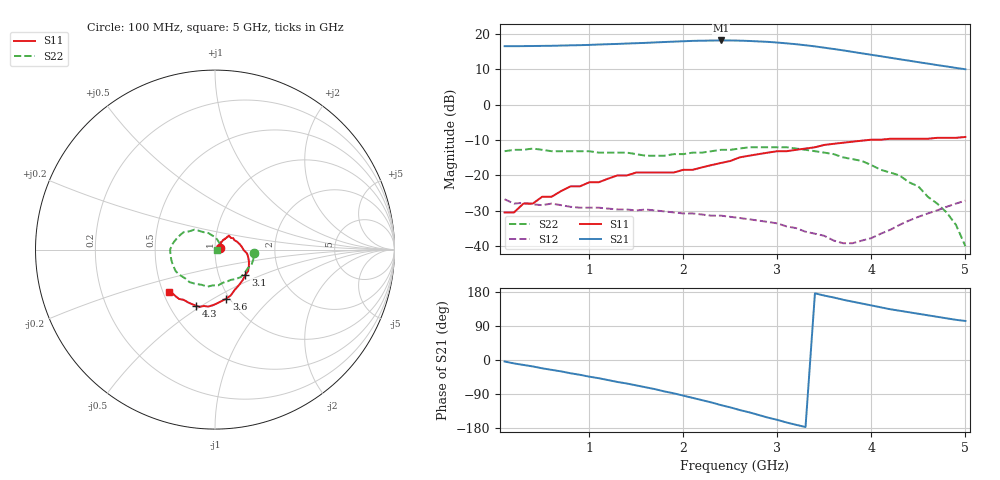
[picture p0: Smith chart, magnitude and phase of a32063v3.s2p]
!  INA-32063  S PARAMETERS
!  Vd = 3 V  LAST UPDATED 04-16-98
# ghz s ma r 50
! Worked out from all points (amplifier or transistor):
!   50 points, 100 MHz to 5 GHz, reference 50 ohm
!   highest |S21| = 18.2 dB at 2.4 GHz (marker M1)
!   |S21| within 3 dB of that: start of sweep to 3.747 GHz
!   unconditionally stable (mu >= 1): start of sweep to end of sweep
!   at 900 MHz: K = 2.07, MAG = 17.1 dB, |S12| = -29.1 dB
!   at 2.6 GHz: K = 2.33, MAG = 18.6 dB, |S12| = -32.0 dB
!   at 5 GHz: K = 3.21, MAG = 10.6 dB, |S12| = -27.1 dB
!   S11 on the Smith chart (normalised r, x): 100 MHz: 1.06, +0.02; 3.1 GHz: 1.34, -0.40; 3.6 GHz: 0.97, -0.57; 4.3 GHz: 0.67, -0.47; 5 GHz: 0.54, -0.29
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0.1  0.03 19.0  6.72 -4.0  0.046 3.0  0.22 -5.0
0.4  0.04 41.0  6.75 -17.0  0.039 -10.0  0.24 -8.0
0.7  0.06 49.0  6.85 -30.0  0.038 -12.0  0.22 -12.0
1  0.08 47.0  7 -44.0  0.035 -11.0  0.22 -25.0
1.4  0.1 46.0  7.32 -62.0  0.033 -15.0  0.21 -47.0
1.7  0.11 41.0  7.59 -77.0  0.032 -19.0  0.19 -68.0
1.8  0.11 38.0  7.69 -83.0  0.031 -20.0  0.19 -77.0
2.1  0.12 26.0  7.98 -100.0  0.029 -25.0  0.21 -101.0
2.3  0.14 13.0  8.06 -112.0  0.027 -29.0  0.22 -120.0
2.4  0.15 6.0  8.09 -119.0  0.027 -31.0  0.23 -128.0
2.6  0.18 -7.0  8.04 -132.0  0.025 -37.0  0.24 -143.0
2.7  0.19 -13.0  7.96 -138.0  0.024 -42.0  0.25 -151.0
2.9  0.21 -26.0  7.73 -152.0  0.022 -51.0  0.25 -166.0
3.1  0.22 -40.0  7.36 -165.0  0.019 -63.0  0.25 180.0
3.4  0.25 -64.0  6.67 176.0  0.015 -86.0  0.22 163.0
3.6  0.28 -77.0  6.13 165.0  0.012 -110.0  0.2 151.0
3.7  0.29 -83.0  5.86 159.0  0.011 -121.0  0.18 146.0
3.9  0.31 -92.0  5.32 149.0  0.012 -142.0  0.16 136.0
4.2  0.33 -105.0  4.61 134.0  0.017 -166.0  0.11 120.0
4.3  0.33 -109.0  4.39 130.0  0.02 -173.0  0.1 112.0
4.8  0.34 -130.0  3.47 110.0  0.036 165.0  0.03 15.0
5  0.35 -137.0  3.17 103.0  0.044 159.0  0.01 -17.0
